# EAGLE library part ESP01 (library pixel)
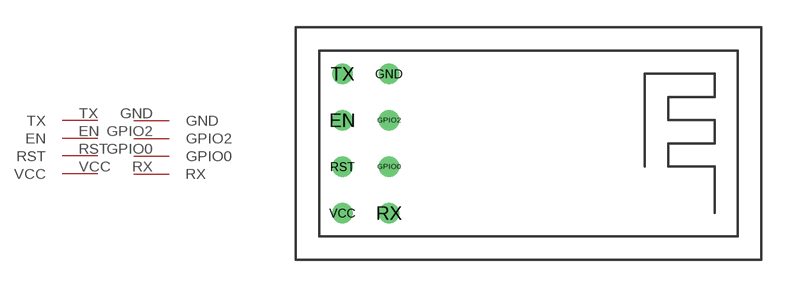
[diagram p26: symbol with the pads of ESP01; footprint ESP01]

Designator prefix -

## ESP01  [ESP01]
EN  EN
GND  GND
GPIO0  GPIO0
GPIO2  GPIO2
RST  RST
RX  RX
TX  TX
VCC  VCC

## Footprint ESP01 (pad centres in mm)
drill 0.6: EN 2.54,7.62; GND 5.08,10.16; GPIO0 5.08,5.08; GPIO2 5.08,7.62; RST 2.54,5.08; RX 5.08,2.54; TX 2.54,10.16; VCC 2.54,2.54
